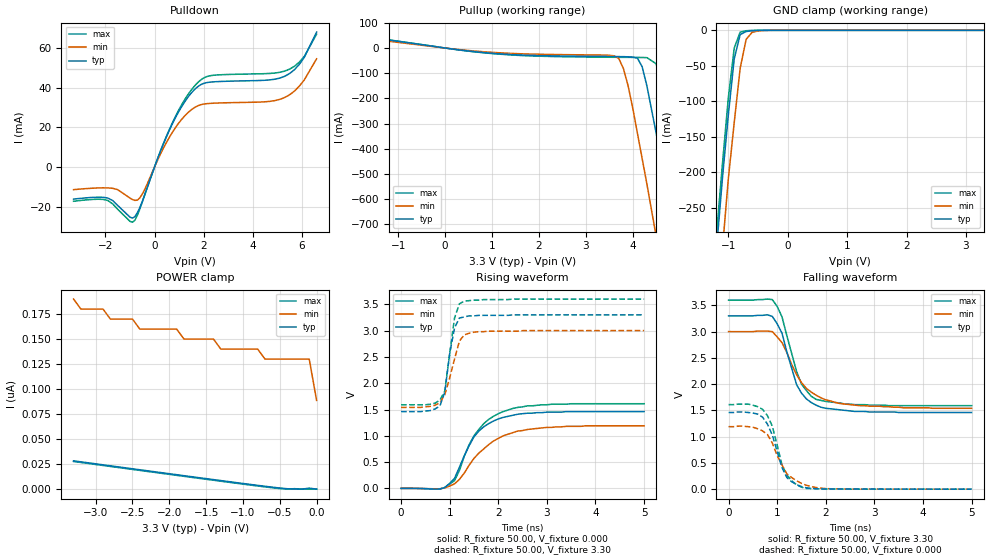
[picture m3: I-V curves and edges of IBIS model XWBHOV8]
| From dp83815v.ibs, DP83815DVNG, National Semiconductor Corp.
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|   Model XWBHOV8
[Model]   XWBHOV8
Model_type   I/O
Polarity   Non-Inverting
Enable   Active-High
Vinl =   0.80V
Vinh =   2.00V
Vmeas =   1.50V
Cref =  20.00pF
Rref = 100.00k
C_comp   5.00pF   5.00pF   5.00pF
[Temperature Range]   25.00   0.14k   0.000
[Voltage Range]   3.30V   3.00V   3.60V
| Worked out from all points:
|   slope of the pulldown table from 0 to 0.495 V, typ, clamps not added: 31.9 ohm
|   slope of the pullup table from 0 to 0.495 V, typ, clamps not added: 41.9 ohm
|   GND clamp passes 1 mA (typ) near -0.64 V on its own axis
|   rising waveform, R_fixture 50.00, V_fixture 0.000: 20-80 % time 549ps typ, 747ps min, 582ps max; typ from 0 V to 1.46 V
|   rising waveform, R_fixture 50.00, V_fixture 3.30: 20-80 % time 177ps typ, 257ps min, 174ps max; typ from 1.46 V to 3.3 V
|   falling waveform, R_fixture 50.00, V_fixture 3.30: 20-80 % time 391ps typ, 587ps min, 384ps max; typ from 3.3 V to 1.46 V
|   falling waveform, R_fixture 50.00, V_fixture 0.000: 20-80 % time 328ps typ, 419ps min, 317ps max; typ from 1.46 V to 0 V
[Pulldown]
| voltage   I(typ)   I(min)   I(max)
-3.3V     -16.25mA   -11.47mA   -17.33mA
-1.9V     -15.71mA   -10.59mA   -16.95mA
-900mV    -25.8mA    -16.46mA   -27.88mA
-700mV    -23.08mA   -16.75mA   -24.35mA
-500mV    -17.42mA   -13.7mA    -17.71mA
700mV     21.07mA    16.93mA    21.53mA
1.2V      32.32mA    25.35mA    33.36mA
1.7V      39.85mA    30.44mA    41.77mA
2.3V      42.79mA    32.06mA    46.05mA
5.3V      45.7mA     35mA       48.32mA
5.9V      51.76mA    40.77mA    52.87mA
6.6V      67.99mA    54.51mA    66.93mA
[Pullup]
| voltage   I(typ)   I(min)   I(max)
-3.3V     66.29mA    12.28mA    73.09mA
-2.5V     60.11mA    48.8mA     62.29mA
3.6V      -33.92mA   -30.83mA   -36.74mA
3.7V      -34.05mA   -41mA      -36.88mA
3.9V      -34.88mA   -150mA     -37.13mA
4.1V      -40.45mA   -340mA     -37.38mA
4.3V      -150mA     -540mA     -38.17mA
4.5V      -340mA     -750mA     -62.71mA
4.9V      -770mA     -1.17A     -430mA
5.1V      -980mA     -1.39A     -640mA
5.3V      -1.2A      -1.6A      -860mA
6.6V      -2.63A     -3.03A     -2.29A
[GND_clamp]
| voltage   I(typ)   I(min)   I(max)
-3.3V     -2.59A     -2.66A     -2.58A
-1.2V     -310mA     -410mA     -290mA
-1.1V     -210mA     -310mA     -190mA
-1V       -120mA     -210mA     -95.83mA
-900mV    -40.16mA   -130mA     -24.89mA
-800mV    -5.96mA    -53.55mA   -2.53mA
-700mV    -1.69mA    -12.88mA   -590uA
-600mV    -600uA     -2.84mA    -110uA
-500mV    -120uA     -970uA     -9.32uA
-200mV    -25.96nA   -6.51uA    -550pA
3.3V      82.67pA    130nA      35.96pA
[POWER_clamp]
| voltage   I(typ)   I(min)   I(max)
-3.3V     28.33nA    190nA      27.7nA
-3.2V     27.34nA    180nA      26.71nA
-2.9V     24.36nA    180nA      23.73nA
-2.8V     23.37nA    170nA      22.74nA
-2.5V     20.4nA     170nA      19.77nA
-2.4V     19.41nA    160nA      18.78nA
-1.9V     14.49nA    160nA      13.85nA
-1.8V     13.5nA     150nA      12.87nA
-800mV    3.84nA     140nA      3.21nA
-700mV    2.92nA     130nA      2.3nA
-100mV    1.07nA     130nA      42.46pA
0V        82.67pA    88.76nA    39.35pA
[Ramp]
| variable   typ   min   max
dV/dt_r   1.84/0.31n   1.64/0.41n   2.01/0.31n
dV/dt_f   1.87/0.28n   1.68/0.41n   2.04/0.27n
R_load = 0.50k
[Rising Waveform]
R_fixture = 50.00
V_fixture = 0.000
V_fixture_min = 0.000
V_fixture_max = 0.000
| time   V(typ)   V(min)   V(max)
0s        98.74uV    85.62uV    110uV
800ps     -11mV      -6.91mV    -13.03mV
900ps     16.11mV    8.88mV     18.29mV
1.1ns     190mV      86.22mV    150mV
1.4ns     810mV      440mV      830mV
1.5ns     980mV      570mV      1V
1.8ns     1.23V      830mV      1.31V
2.1ns     1.35V      1V         1.46V
3ns       1.45V      1.16V      1.59V
5ns       1.46V      1.19V      1.61V
[Rising Waveform]
R_fixture = 50.00
V_fixture = 3.30
V_fixture_min = 3.00
V_fixture_max = 3.60
| time   V(typ)   V(min)   V(max)
0s        1.46V      1.54V      1.59V
600ps     1.48V      1.56V      1.6V
800ps     1.57V      1.63V      1.68V
900ps     1.83V      1.78V      1.85V
1ns       2.56V      2.1V       2.56V
1.1ns     3.05V      2.46V      3.24V
1.2ns     3.24V      2.8V       3.51V
1.3ns     3.26V      2.92V      3.56V
1.8ns     3.29V      2.99V      3.59V
5ns       3.3V       3V         3.6V
[Falling Waveform]
R_fixture = 50.00
V_fixture = 3.30
V_fixture_min = 3.00
V_fixture_max = 3.60
| time   V(typ)   V(min)   V(max)
0s        3.3V       3V         3.6V
900ps     3.29V      3V         3.61V
1.1ns     2.97V      2.79V      3.28V
1.4ns     1.99V      2.18V      2.24V
1.5ns     1.83V      2.03V      2V
1.7ns     1.65V      1.85V      1.77V
1.8ns     1.6V       1.79V      1.71V
2.2ns     1.52V      1.65V      1.65V
2.7ns     1.48V      1.59V      1.61V
5ns       1.46V      1.54V      1.59V
[Falling Waveform]
R_fixture = 50.00
V_fixture = 0.000
V_fixture_min = 0.000
V_fixture_max = 0.000
| time   V(typ)   V(min)   V(max)
0s        1.46V      1.19V      1.61V
400ps     1.46V      1.19V      1.62V
700ps     1.37V      1.11V      1.52V
800ps     1.24V      1.04V      1.4V
900ps     1.03V      880mV      1.2V
1.1ns     410mV      460mV      460mV
1.2ns     220mV      290mV      270mV
1.5ns     49.86mV    110mV      37.33mV
2.1ns     3.65mV     7.32mV     3.86mV
5ns       56.94uV    66.42uV    49.59uV
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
